|   Microchip Technology Inc.
|   PolarFire IBIS Model
[IBIS ver]   5.0
[File name]   polarfire_dio.ibs
[File Rev]   1.4
[Date]   Tue Jun 20 2023
[Source] Simulated Models ONLY.
   All data is based on Spice simulation. All performed at Microchip Technology Inc..
[Notes]  IBIS file for dedicated I/O Standards.
   The package parasitics of various package types are given.
   Uncomment the appropriate package before simulations.
   Revision History:
   Rev 1.4: 20-Jun-2023
   - Updated Vinl and Vinh values of LVPECL_33,MIPI_25,MIPI_33 receivers
   Rev 1.3: 23-May-2022
   - REFCLK buffers mapped to the VDD_XCVR_CLK supply in [Pin Mapping] section
   - Added MPF050 device with RLC package data in [Package] section
   - Added RLC package type of FCG784N for MPF300T device
   - Update RLC package data for 100T/200T/300T/500T devices
   Rev 1.2: 20-Sept-2021
   - Addition of LVDS ODT models
   Rev 1.1: 29-oct-2018
   - Fixed Power Clamp and Gnd Clamp data of standards
   LVTTL_33_ODT-OFF_HYST-OFF_refclk and LVCMOS25_25_ODT-75_HYST-ON_refclk
   - Added one supply pin in [pin] section
   - Added pin description in [Pin] section
   - Added [Pin Mapping] section
[Disclaimer] This information is for board design considerations.
   Simulation based V/I curves contained in this model file are
   considered preliminary until verified against bench
   measurements. Maximum currents may vary from part to part but
   should not exceed maximum I/V curves provided in this model file.
[Copyright]  (c) 2023, Microchip Technology Inc., All Rights Reserved.
| ADDITIONAL NOTES
| The naming conventions used in the signal_name/model_name are as follows:
| HYST-#  - Hysteresis setting,OFF or ON represented by #
| ODT-#   - Series on-die termination, impedance value represented by #
| #_I   - Refers to input models ,  model name represented by #
| #_O   - Refers to output models , model name represented by #
| #_IO   - Refers to Input/Output models,  model name represented by #
| IBIS MODEL CHECKLIST
| Microchip Technology Inc. is dedicated to releasing quality IBIS models to customers.
| The following items have been
| verified for this IBIS model before release:
| 1)  Checked IBIS model by the golden parser ibischk5 [Complete]
| 2)  Ensured no errors reported by golden parser
|   for the IBIS model [Complete]
| 3)  Defined Vinl and Vinh for receivers [Complete]
| 4)  Defined Standard Load and Vmeas values for drivers [Complete]
| 5)  Defined overshoots for drivers and receivers [NA]
| 6)  Validated Ramp Values[]
| 7)  Defined V-T Tables for all output drivers [Complete]
| 8)  Validated [Diff Pins] [NA]
| 9)  Verified Package Parasitics [Complete]
| 10) Defined Standard Load Parameters and Specifications
|   for waveforms [Complete]
| 11) Defined and Validate Pin mappings [Complete]
| 12) Verified Ccomp Value []
| 13) Visually Inspected I-V Curves and V-T Tables  [Complete]
| 14) Presented Typ/Min/Max Values in the correct order for
|   all tables and parameters [Complete]
| 15) Simulated all output models with standard load and
|   switching through Vmeas [Complete]
| 16) Simulated all receiver models  [Complete]
| 17) Validated Models selectors. [Complete]
| 18) Visually inspected Spice and IBIS correlation for
|   a) Typical VT Curves [Complete]
|   b) Minimum VT Curves [Complete]
|   c) Maximum VT Curves [Complete]
| 19) Visually inspected Silicon and IBIS correlation
|   a) Typical IV Pull UP/ Pull Down Curves []
|   b) Minimum IV Pull UP/ Pull Down Curves []
|   c) Maximum IV Pull UP/ Pull Down Curves []
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[Component]   PolarFire
[Manufacturer]   Microchip Technology Inc.
[Package]
|   typ   min   max
|MPF050T/TL/TLS/TS
|R_pkg   0.204   NA   NA   | MPF050T/TL/TLS/TS-FCSG325
|L_pkg   1.608nH   NA   NA   | MPF050T/TL/TLS/TS-FCSG325
|C_pkg   0.803pF   NA   NA   | MPF050T/TL/TLS/TS-FCSG325
|R_pkg   0.570   NA   NA   | MPF050T/TL/TLS/TS-FCVG484
|L_pkg   3.557nH   NA   NA   | MPF050T/TL/TLS/TS-FCVG484
|C_pkg   1.663pF   NA   NA   | MPF050T/TL/TLS/TS-FCVG484
|MPF100T/TL/TLS/TS
|R_pkg   0.253   NA   NA   | MPF100T/TL/TLS/TS-FCSG325
|L_pkg   1.920nH   NA   NA   | MPF100T/TL/TLS/TS-FCSG325
|C_pkg   0.703pF   NA   NA   | MPF100T/TL/TLS/TS-FCSG325
|R_pkg   0.628   NA   NA   | MPF100T/TL/TLS/TS-FCG484
|L_pkg   4.759nH   NA   NA   | MPF100T/TL/TLS/TS-FCG484
|C_pkg   2.176pF   NA   NA   | MPF100T/TL/TLS/TS-FCG484
|R_pkg   0.355   NA   NA   | MPF100T/TL/TLS/TS-FCVG484
|L_pkg   2.999nH   NA   NA   | MPF100T/TL/TLS/TS-FCVG484
|C_pkg   1.416pF   NA   NA   | MPF100T/TL/TLS/TS-FCVG484
|MPF200T/TL/TLS/TS
|R_pkg   0.316   NA   NA   | MPF200T/TL/TLS/TS-FCSG325
|L_pkg   2.423nH   NA   NA   | MPF200T/TL/TLS/TS-FCSG325
|C_pkg   0.844pF   NA   NA   | MPF200T/TL/TLS/TS-FCSG325
|R_pkg   0.518   NA   NA   | MPF200T/TL/TLS/TS-FCG484
|L_pkg   4.022nH   NA   NA   | MPF200T/TL/TLS/TS-FCG484
|C_pkg   1.858pF   NA   NA   | MPF200T/TL/TLS/TS-FCG484
|R_pkg   0.603   NA   NA   | MPF200T/TL/TLS/TS-FCVG484
|L_pkg   3.944nH   NA   NA   | MPF200T/TL/TLS/TS-FCVG484
|C_pkg   1.558pF   NA   NA   | MPF200T/TL/TLS/TS-FCVG484
|R_pkg   0.374   NA   NA   | MPF200T/TL/TLS/TS-FCSG536
|L_pkg   3.833nH   NA   NA   | MPF200T/TL/TLS/TS-FCSG536
|C_pkg   0.996pF   NA   NA   | MPF200T/TL/TLS/TS-FCSG536
|R_pkg   0.444   NA   NA   | MPF200T/TL/TLS/TS-FCG784
|L_pkg   3.672nH   NA   NA   | MPF200T/TL/TLS/TS-FCG784
|C_pkg   1.699pF   NA   NA   | MPF200T/TL/TLS/TS-FCG784
|MPF300T/TL/TLS/TS
|R_pkg   0.228   NA   NA   | MPF300T/TL/TLS/TS-FCG484
|L_pkg   2.178nH   NA   NA   | MPF300T/TL/TLS/TS-FCG484
|C_pkg   1.408pF   NA   NA   | MPF300T/TL/TLS/TS-FCG484
|R_pkg   0.661   NA   NA   | MPF300T/TL/TLS/TS-FCVG484
|L_pkg   4.585nH   NA   NA   | MPF300T/TL/TLS/TS-FCVG484
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R_pkg   0.735   NA   NA   | MPF300T/TL/TLS/TS-FCG1152
L_pkg   5.088nH   NA   NA   | MPF300T/TL/TLS/TS-FCG1152
C_pkg   2.163pF   NA   NA   | MPF300T/TL/TLS/TS-FCG1152
|MPF500T/TL/TLS/TS
|R_pkg   0.522   NA   NA   | MPF500T/TL/TLS/TS-FCG784
|L_pkg   3.540nH   NA   NA   | MPF500T/TL/TLS/TS-FCG784
|C_pkg   1.604pF   NA   NA   | MPF500T/TL/TLS/TS-FCG784
|R_pkg   0.594   NA   NA   | MPF500T/TL/TLS/TS-FCG1152
|L_pkg   3.914nH   NA   NA   | MPF500T/TL/TLS/TS-FCG1152
|C_pkg   1.587pF   NA   NA   | MPF500T/TL/TLS/TS-FCG1152
| End Header
| The PIN numbers given below are examples. They do not correspond to
| device pin numbers.
[Pin]   signal_name   model_name   R_pin   L_pin   C_pin
| SPI signals
1   sc_spi_sck   LVCMOS_iobuf_dio
2   sc_spi_ss   LVCMOS_iobuf_dio
3   sc_spi_sdo   LVCMOS_obuf_dio
| JTAG signals
4   jtag_tdo   LVCMOS_obuf_dio
5   jtag_tms   LVCMOS_ibuf_pullup_dio
6   jtag_tdi   LVCMOS_ibuf_pullup_dio
7   jtag_tck   LVCMOS_ibuf_dio
8   jtag_trstb   LVCMOS_ibuf_pullup_dio
| Device Reset (DEVRST_N)
9   devrst_b   LVCMOS_ibuf_pullup_dio
| UNUSED
10   sc_exit_flash_freeze   LVCMOS_ibuf_pullup_dio
| SPI signals
11   sc_spi_sdi   LVCMOS_ibuf_dio
12   sc_io_cfg_interface   LVCMOS_ibuf_dio
13   sc_io_cfg_flash   LVCMOS_ibuf_dio
| SERDES REFCLK
14   ref_clk   ref_clk_inputs
| Power Supplies
15   VDDI   POWER
16   VDD_XCVR_CLK   POWER
17   VSS   GND
| SERDES REFCLK_DIFF
18P   ref_clk_diff_ODT_OFF_P   ref_clk_inputs_DIFF_ODT_OFF
18N   ref_clk_diff_ODT_OFF_N   ref_clk_inputs_DIFF_ODT_OFF
19P   ref_clk_diff_ODT_ON_33_P   ref_clk_inputs_diff_ODT_ON_33
19N   ref_clk_diff_ODT_ON_33_N   ref_clk_inputs_diff_ODT_ON_33
20P   ref_clk_diff_ODT_ON_25_P   ref_clk_inputs_diff_ODT_ON_25
20N   ref_clk_diff_ODT_ON_25_N   ref_clk_inputs_diff_ODT_ON_25
[Pin Mapping]   pulldown_ref   pullup_ref   gnd_clamp_ref   power_clamp_ref ext_ref
1   VSS   VDDI   VSS   VDDI
2   VSS   VDDI   VSS   VDDI
3   VSS   VDDI   VSS   VDDI
4   VSS   VDDI   VSS   VDDI
5   VSS   VDDI   VSS   VDDI
6   VSS   VDDI   VSS   VDDI
7   VSS   VDDI   VSS   VDDI
8   VSS   VDDI   VSS   VDDI
9   VSS   VDDI   VSS   VDDI
10   VSS   VDDI   VSS   VDDI
11   VSS   VDDI   VSS   VDDI
12   VSS   VDDI   VSS   VDDI
13   VSS   VDDI   VSS   VDDI
14   VSS   VDD_XCVR_CLK   VSS   VDD_XCVR_CLK
15   NC   VDDI
16   NC   VDD_XCVR_CLK
17   VSS   NC
18P   VSS   VDD_XCVR_CLK   VSS   VDD_XCVR_CLK
18N   VSS   VDD_XCVR_CLK   VSS   VDD_XCVR_CLK
19P   VSS   VDD_XCVR_CLK   VSS   VDD_XCVR_CLK
19N   VSS   VDD_XCVR_CLK   VSS   VDD_XCVR_CLK
20P   VSS   VDD_XCVR_CLK   VSS   VDD_XCVR_CLK
20N   VSS   VDD_XCVR_CLK   VSS   VDD_XCVR_CLK
[Diff Pin]   inv_pin   vdiff   tdelay_typ   tdelay_min   tdelay_max
18P   18N   100mV   0   0   0
19P   19N   100mV   0   0   0
20P   20N   100mV   0   0   0
[Series Pin Mapping]   pin_2   model_name   function_table_group
19P   19N   ODT_33_TERM_100
20P   20N   ODT_25_TERM_100
|   Model Selector
[Model Selector]   LVCMOS_iobuf_dio
LVCMOS_33_HYST-ON_DIO_IO   3.3V I/O hysteresis ON
LVCMOS_25_HYST-ON_DIO_IO   2.5V I/O hysteresis ON
LVCMOS_18_HYST-ON_DIO_IO   1.8V I/O hysteresis ON
[Model Selector]   LVCMOS_obuf_dio
LVCMOS_33_HYST-OFF_DIO_O   3.3V Output hysteresis OFF
LVCMOS_25_HYST-OFF_DIO_O   2.5V Output hysteresis OFF
LVCMOS_18_HYST-OFF_DIO_O   1.8V Output hysteresis OFF
[Model Selector]   LVCMOS_ibuf_pullup_dio
LVCMOS_33_PM_HYST-ON_DIO_I   3.3V Input weak pullup hysteresis ON
LVCMOS_25_PM_HYST-ON_DIO_I   2.5V Input weak pullup hysteresis ON
LVCMOS_18_PM_DIO_I   1.8V Input weak pullup
[Model Selector]   LVCMOS_ibuf_dio
LVCMOS_33_HYST-ON_DIO_I   3.3V Input hysteresis ON
LVCMOS_25_HYST-ON_DIO_I   2.5V Input hysteresis ON
LVCMOS_18_DIO_I   1.8V Input
[Model Selector]   ref_clk_inputs
LVTTL_33_ODT-OFF_HYST-ON_refclk   3.3V LVTTL Standard
LVTTL_25_ODT-OFF_HYST-ON_refclk   2.5V LVTTL Standard
LVTTL_33_ODT-75_HYST-ON_refclk   3.3V LVTTL Standard
LVTTL_25_ODT-75_HYST-ON_refclk   2.5V LVTTL Standard
LVTTL_33_ODT-150_HYST-ON_refclk   3.3V LVTTL Standard
LVTTL_25_ODT-150_HYST-ON_refclk   2.5V LVTTL Standard
LVTTL_33_ODT-OFF_HYST-OFF_refclk   3.3V LVTTL Standard
LVTTL_25_ODT-OFF_HYST-OFF_refclk   2.5V LVTTL Standard
LVTTL_33_ODT-75_HYST-OFF_refclk   3.3V LVTTL Standard
LVTTL_25_ODT-75_HYST-OFF_refclk   2.5V LVTTL Standard
LVTTL_33_ODT-150_HYST-OFF_refclk   3.3V LVTTL Standard
LVTTL_25_ODT-150_HYST-OFF_refclk   2.5V LVTTL Standard
LVCMOS33_33_ODT-OFF_HYST-ON_refclk   3.3V LVCMOS33 Standard
LVCMOS33_25_ODT-OFF_HYST-ON_refclk   2.5V LVCMOS33 Standard
LVCMOS33_33_ODT-75_HYST-ON_refclk   3.3V LVCMOS33 Standard
LVCMOS33_25_ODT-75_HYST-ON_refclk   2.5V LVCMOS33 Standard
LVCMOS33_33_ODT-150_HYST-ON_refclk   3.3V LVCMOS33 Standard
LVCMOS33_25_ODT-150_HYST-ON_refclk   2.5V LVCMOS33 Standard
LVCMOS33_33_ODT-OFF_HYST-OFF_refclk   3.3V LVCMOS33 Standard
LVCMOS33_25_ODT-OFF_HYST-OFF_refclk   2.5V LVCMOS33 Standard
LVCMOS33_33_ODT-75_HYST-OFF_refclk   3.3V LVCMOS33 Standard
LVCMOS33_25_ODT-75_HYST-OFF_refclk   2.5V LVCMOS33 Standard
LVCMOS33_33_ODT-150_HYST-OFF_refclk   3.3V LVCMOS33 Standard
LVCMOS33_25_ODT-150_HYST-OFF_refclk   2.5V LVCMOS33 Standard
LVCMOS25_33_ODT-OFF_HYST-ON_refclk   3.3V LVCMOS25 Standard
LVCMOS25_25_ODT-OFF_HYST-ON_refclk   2.5V LVCMOS25 Standard
LVCMOS25_33_ODT-75_HYST-ON_refclk   3.3V LVCMOS25 Standard
LVCMOS25_25_ODT-75_HYST-ON_refclk   2.5V LVCMOS25 Standard
LVCMOS25_33_ODT-150_HYST-ON_refclk   3.3V LVCMOS25 Standard
LVCMOS25_25_ODT-150_HYST-ON_refclk   2.5V LVCMOS25 Standard
LVCMOS25_33_ODT-OFF_HYST-OFF_refclk   3.3V LVCMOS25 Standard
LVCMOS25_25_ODT-OFF_HYST-OFF_refclk   2.5V LVCMOS25 Standard
LVCMOS25_33_ODT-75_HYST-OFF_refclk   3.3V LVCMOS25 Standard
LVCMOS25_25_ODT-75_HYST-OFF_refclk   2.5V LVCMOS25 Standard
LVCMOS25_33_ODT-150_HYST-OFF_refclk   3.3V LVCMOS25 Standard
LVCMOS25_25_ODT-150_HYST-OFF_refclk   2.5V LVCMOS25 Standard
LVCMOS18_18_ODT-OFF_HYST-ON_refclk   1.8V LVCMOS18 Standard
LVCMOS18_25_ODT-OFF_HYST-ON_refclk   2.5V LVCMOS18 Standard
LVCMOS18_18_ODT-75_HYST-ON_refclk   1.8V LVCMOS18 Standard
LVCMOS18_25_ODT-75_HYST-ON_refclk   2.5V LVCMOS18 Standard
LVCMOS18_18_ODT-150_HYST-ON_refclk   1.8V LVCMOS18 Standard
LVCMOS18_25_ODT-150_HYST-ON_refclk   2.5V LVCMOS18 Standard
LVCMOS18_18_ODT-OFF_HYST-OFF_refclk   1.8V LVCMOS18 Standard
LVCMOS18_25_ODT-OFF_HYST-OFF_refclk   2.5V LVCMOS18 Standard
LVCMOS18_18_ODT-75_HYST-OFF_refclk   1.8V LVCMOS18 Standard
LVCMOS18_25_ODT-75_HYST-OFF_refclk   2.5V LVCMOS18 Standard
LVCMOS18_18_ODT-150_HYST-OFF_refclk   1.8V LVCMOS18 Standard
LVCMOS18_25_ODT-150_HYST-OFF_refclk   2.5V LVCMOS18 Standard
SSTL25I_25_ODT-OFF_HYST-ON_refclk   2.5V SSTL25I Standard
SSTL25I_25_ODT-OFF_HYST-OFF_refclk   2.5V SSTL25I Standard
SSTL25II_25_ODT-OFF_HYST-ON_refclk   2.5V SSTL25II Standard
SSTL25II_25_ODT-OFF_HYST-OFF_refclk   2.5V SSTL25II Standard
SSTL18I_25_ODT-OFF_HYST-ON_refclk   2.5V SSTL18I Standard
SSTL18I_25_ODT-OFF_HYST-OFF_refclk   2.5V SSTL18I Standard
SSTL18II_25_ODT-OFF_HYST-ON_refclk   2.5V SSTL18II Standard
SSTL18II_25_ODT-OFF_HYST-OFF_refclk   2.5V SSTL18II Standard
SSTL25DI_25_ODT-OFF_HYST-ON_N_refclk   2.5V SSTL25DI Standard
SSTL25DI_25_ODT-OFF_HYST-ON_P_refclk   2.5V SSTL25DI Standard
SSTL25DI_25_ODT-OFF_HYST-OFF_N_refclk   2.5V SSTL25DI Standard
SSTL25DI_25_ODT-OFF_HYST-OFF_P_refclk   2.5V SSTL25DI Standard
SSTL25DII_25_ODT-OFF_HYST-ON_N_refclk   2.5V SSTL25DII Standard
SSTL25DII_25_ODT-OFF_HYST-ON_P_refclk   2.5V SSTL25DII Standard
SSTL25DII_25_ODT-OFF_HYST-OFF_N_refclk   2.5V SSTL25DII Standard
SSTL25DII_25_ODT-OFF_HYST-OFF_P_refclk   2.5V SSTL25DII Standard
SSTL18DI_25_ODT-OFF_HYST-ON_N_refclk   2.5V SSTL18DI Standard
SSTL18DI_25_ODT-OFF_HYST-ON_P_refclk   2.5V SSTL18DI Standard
SSTL18DI_25_ODT-OFF_HYST-OFF_N_refclk   2.5V SSTL18DI Standard
SSTL18DI_25_ODT-OFF_HYST-OFF_P_refclk   2.5V SSTL18DI Standard
SSTL18DII_25_ODT-OFF_HYST-ON_N_refclk   2.5V SSTL18DII Standard
SSTL18DII_25_ODT-OFF_HYST-ON_P_refclk   2.5V SSTL18DII Standard
SSTL18DII_25_ODT-OFF_HYST-OFF_N_refclk   2.5V SSTL18DII Standard
SSTL18DII_25_ODT-OFF_HYST-OFF_P_refclk   2.5V SSTL18DII Standard
HSUL18I_25_ODT-OFF_HYST-ON_refclk   2.5V HSUL18I Standard
HSUL18I_25_ODT-OFF_HYST-OFF_refclk   2.5V HSUL18I Standard
HSUL18II_25_ODT-OFF_HYST-ON_refclk   2.5V HSUL18II Standard
HSUL18II_25_ODT-OFF_HYST-OFF_refclk   2.5V HSUL18II Standard
HSUL18DI_25_ODT-OFF_HYST-ON_N_refclk   2.5V HSUL18DI Standard
HSUL18DI_25_ODT-OFF_HYST-ON_P_refclk   2.5V HSUL18DI Standard
HSUL18DI_25_ODT-OFF_HYST-OFF_N_refclk   2.5V HSUL18DI Standard
HSUL18DI_25_ODT-OFF_HYST-OFF_P_refclk   2.5V HSUL18DI Standard
HSUL18DII_25_ODT-OFF_HYST-ON_N_refclk   2.5V HSUL18DII Standard
HSUL18DII_25_ODT-OFF_HYST-ON_P_refclk   2.5V HSUL18DII Standard
HSUL18DII_25_ODT-OFF_HYST-OFF_N_refclk   2.5V HSUL18DII Standard
HSUL18DII_25_ODT-OFF_HYST-OFF_P_refclk   2.5V HSUL18DII Standard
[Model Selector]   ref_clk_inputs_DIFF_ODT_OFF
LVDS_33_ODT-OFF_HYST-ON_N_refclk   3.3V LVDS Standard
LVDS_33_ODT-OFF_HYST-ON_P_refclk   3.3V LVDS Standard
LVDS_25_ODT-OFF_HYST-ON_N_refclk   2.5V LVDS Standard
LVDS_25_ODT-OFF_HYST-ON_P_refclk   2.5V LVDS Standard
LVDS_33_ODT-OFF_HYST-OFF_N_refclk   3.3V LVDS Standard
LVDS_33_ODT-OFF_HYST-OFF_P_refclk   3.3V LVDS Standard
LVDS_25_ODT-OFF_HYST-OFF_N_refclk   2.5V LVDS Standard
LVDS_25_ODT-OFF_HYST-OFF_P_refclk   2.5V LVDS Standard
RSDS_33_ODT-OFF_HYST-ON_N_refclk   3.3V RSDS Standard
RSDS_33_ODT-OFF_HYST-ON_P_refclk   3.3V RSDS Standard
RSDS_25_ODT-OFF_HYST-ON_N_refclk   2.5V RSDS Standard
RSDS_25_ODT-OFF_HYST-ON_P_refclk   2.5V RSDS Standard
RSDS_33_ODT-OFF_HYST-OFF_N_refclk   3.3V RSDS Standard
RSDS_33_ODT-OFF_HYST-OFF_P_refclk   3.3V RSDS Standard
RSDS_25_ODT-OFF_HYST-OFF_N_refclk   2.5V RSDS Standard
RSDS_25_ODT-OFF_HYST-OFF_P_refclk   2.5V RSDS Standard
MINILVDS_33_ODT-OFF_HYST-ON_N_refclk   3.3V MINILVDS Standard
MINILVDS_33_ODT-OFF_HYST-ON_P_refclk   3.3V MINILVDS Standard
MINILVDS_25_ODT-OFF_HYST-ON_N_refclk   2.5V MINILVDS Standard
MINILVDS_25_ODT-OFF_HYST-ON_P_refclk   2.5V MINILVDS Standard
MINILVDS_33_ODT-OFF_HYST-OFF_N_refclk   3.3V MINILVDS Standard
MINILVDS_33_ODT-OFF_HYST-OFF_P_refclk   3.3V MINILVDS Standard
MINILVDS_25_ODT-OFF_HYST-OFF_N_refclk   2.5V MINILVDS Standard
MINILVDS_25_ODT-OFF_HYST-OFF_P_refclk   2.5V MINILVDS Standard
SUBLVDS_33_ODT-OFF_HYST-ON_N_refclk   3.3V SUBLVDS Standard
SUBLVDS_33_ODT-OFF_HYST-ON_P_refclk   3.3V SUBLVDS Standard
SUBLVDS_25_ODT-OFF_HYST-ON_N_refclk   2.5V SUBLVDS Standard
SUBLVDS_25_ODT-OFF_HYST-ON_P_refclk   2.5V SUBLVDS Standard
SUBLVDS_33_ODT-OFF_HYST-OFF_N_refclk   3.3V SUBLVDS Standard
SUBLVDS_33_ODT-OFF_HYST-OFF_P_refclk   3.3V SUBLVDS Standard
SUBLVDS_25_ODT-OFF_HYST-OFF_N_refclk   2.5V SUBLVDS Standard
SUBLVDS_25_ODT-OFF_HYST-OFF_P_refclk   2.5V SUBLVDS Standard
PPDS_33_ODT-OFF_HYST-ON_N_refclk   3.3V PPDS Standard
PPDS_33_ODT-OFF_HYST-ON_P_refclk   3.3V PPDS Standard
PPDS_25_ODT-OFF_HYST-ON_N_refclk   2.5V PPDS Standard
PPDS_25_ODT-OFF_HYST-ON_P_refclk   2.5V PPDS Standard
PPDS_33_ODT-OFF_HYST-OFF_N_refclk   3.3V PPDS Standard
PPDS_33_ODT-OFF_HYST-OFF_P_refclk   3.3V PPDS Standard
PPDS_25_ODT-OFF_HYST-OFF_N_refclk   2.5V PPDS Standard
PPDS_25_ODT-OFF_HYST-OFF_P_refclk   2.5V PPDS Standard
SLVS_33_ODT-OFF_HYST-ON_N_refclk   3.3V SLVS Standard
SLVS_33_ODT-OFF_HYST-ON_P_refclk   3.3V SLVS Standard
SLVS_25_ODT-OFF_HYST-ON_N_refclk   2.5V SLVS Standard
SLVS_25_ODT-OFF_HYST-ON_P_refclk   2.5V SLVS Standard
SLVS_33_ODT-OFF_HYST-OFF_N_refclk   3.3V SLVS Standard
SLVS_33_ODT-OFF_HYST-OFF_P_refclk   3.3V SLVS Standard
SLVS_25_ODT-OFF_HYST-OFF_N_refclk   2.5V SLVS Standard
SLVS_25_ODT-OFF_HYST-OFF_P_refclk   2.5V SLVS Standard
HCSL_33_ODT-OFF_HYST-ON_N_refclk   3.3V HCSL Standard
HCSL_33_ODT-OFF_HYST-ON_P_refclk   3.3V HCSL Standard
HCSL_25_ODT-OFF_HYST-ON_N_refclk   2.5V HCSL Standard
HCSL_25_ODT-OFF_HYST-ON_P_refclk   2.5V HCSL Standard
HCSL_33_ODT-OFF_HYST-OFF_N_refclk   3.3V HCSL Standard
HCSL_33_ODT-OFF_HYST-OFF_P_refclk   3.3V HCSL Standard
HCSL_25_ODT-OFF_HYST-OFF_N_refclk   2.5V HCSL Standard
HCSL_25_ODT-OFF_HYST-OFF_P_refclk   2.5V HCSL Standard
MLVDS_33_ODT-OFF_HYST-ON_N_refclk   3.3V MLVDS Standard
MLVDS_33_ODT-OFF_HYST-ON_P_refclk   3.3V MLVDS Standard
MLVDS_25_ODT-OFF_HYST-ON_N_refclk   2.5V MLVDS Standard
MLVDS_25_ODT-OFF_HYST-ON_P_refclk   2.5V MLVDS Standard
MLVDS_33_ODT-OFF_HYST-OFF_N_refclk   3.3V MLVDS Standard
MLVDS_33_ODT-OFF_HYST-OFF_P_refclk   3.3V MLVDS Standard
MLVDS_25_ODT-OFF_HYST-OFF_N_refclk   2.5V MLVDS Standard
MLVDS_25_ODT-OFF_HYST-OFF_P_refclk   2.5V MLVDS Standard
LVPECL_33_ODT-OFF_HYST-ON_N_refclk   3.3V LVPECL Standard
LVPECL_33_ODT-OFF_HYST-ON_P_refclk   3.3V LVPECL Standard
LVPECL_33_ODT-OFF_HYST-OFF_N_refclk   3.3V LVPECL Standard
LVPECL_33_ODT-OFF_HYST-OFF_P_refclk   3.3V LVPECL Standard
MIPI_25_ODT-OFF_HYST-ON_N_refclk   2.5V MIPI Standard
MIPI_25_ODT-OFF_HYST-ON_P_refclk   2.5V MIPI Standard
MIPI_33_ODT-OFF_HYST-ON_N_refclk   3.3V MIPI Standard
MIPI_33_ODT-OFF_HYST-ON_P_refclk   3.3V MIPI Standard
MIPI_25_ODT-OFF_HYST-OFF_N_refclk   2.5V MIPI Standard
MIPI_25_ODT-OFF_HYST-OFF_P_refclk   2.5V MIPI Standard
MIPI_33_ODT-OFF_HYST-OFF_N_refclk   3.3V MIPI Standard
MIPI_33_ODT-OFF_HYST-OFF_P_refclk   3.3V MIPI Standard
[Model Selector]   ref_clk_inputs_diff_ODT_ON_33
LVDS_33_ODT-OFF_HYST-ON_N_refclk   3.3V LVDS Standard
LVDS_33_ODT-OFF_HYST-ON_P_refclk   3.3V LVDS Standard
LVDS_33_ODT-OFF_HYST-OFF_N_refclk   3.3V LVDS Standard
LVDS_33_ODT-OFF_HYST-OFF_P_refclk   3.3V LVDS Standard
RSDS_33_ODT-OFF_HYST-ON_N_refclk   3.3V RSDS Standard
RSDS_33_ODT-OFF_HYST-ON_P_refclk   3.3V RSDS Standard
RSDS_33_ODT-OFF_HYST-OFF_N_refclk   3.3V RSDS Standard
RSDS_33_ODT-OFF_HYST-OFF_P_refclk   3.3V RSDS Standard
MINILVDS_33_ODT-OFF_HYST-ON_N_refclk   3.3V MINILVDS Standard
MINILVDS_33_ODT-OFF_HYST-ON_P_refclk   3.3V MINILVDS Standard
MINILVDS_33_ODT-OFF_HYST-OFF_N_refclk   3.3V MINILVDS Standard
MINILVDS_33_ODT-OFF_HYST-OFF_P_refclk   3.3V MINILVDS Standard
SUBLVDS_33_ODT-OFF_HYST-ON_N_refclk   3.3V SUBLVDS Standard
SUBLVDS_33_ODT-OFF_HYST-ON_P_refclk   3.3V SUBLVDS Standard
SUBLVDS_33_ODT-OFF_HYST-OFF_N_refclk   3.3V SUBLVDS Standard
SUBLVDS_33_ODT-OFF_HYST-OFF_P_refclk   3.3V SUBLVDS Standard
PPDS_33_ODT-OFF_HYST-ON_N_refclk   3.3V PPDS Standard
PPDS_33_ODT-OFF_HYST-ON_P_refclk   3.3V PPDS Standard
PPDS_33_ODT-OFF_HYST-OFF_N_refclk   3.3V PPDS Standard
PPDS_33_ODT-OFF_HYST-OFF_P_refclk   3.3V PPDS Standard
SLVS_33_ODT-OFF_HYST-ON_N_refclk   3.3V SLVS Standard
SLVS_33_ODT-OFF_HYST-ON_P_refclk   3.3V SLVS Standard
SLVS_33_ODT-OFF_HYST-OFF_N_refclk   3.3V SLVS Standard
SLVS_33_ODT-OFF_HYST-OFF_P_refclk   3.3V SLVS Standard
HCSL_33_ODT-OFF_HYST-ON_N_refclk   3.3V HCSL Standard
HCSL_33_ODT-OFF_HYST-ON_P_refclk   3.3V HCSL Standard
HCSL_33_ODT-OFF_HYST-OFF_N_refclk   3.3V HCSL Standard
HCSL_33_ODT-OFF_HYST-OFF_P_refclk   3.3V HCSL Standard
MLVDS_33_ODT-OFF_HYST-ON_N_refclk   3.3V MLVDS Standard
MLVDS_33_ODT-OFF_HYST-ON_P_refclk   3.3V MLVDS Standard
MLVDS_33_ODT-OFF_HYST-OFF_N_refclk   3.3V MLVDS Standard
MLVDS_33_ODT-OFF_HYST-OFF_P_refclk   3.3V MLVDS Standard
LVPECL_33_ODT-OFF_HYST-ON_N_refclk   3.3V LVPECL Standard
LVPECL_33_ODT-OFF_HYST-ON_P_refclk   3.3V LVPECL Standard
LVPECL_33_ODT-OFF_HYST-OFF_N_refclk   3.3V LVPECL Standard
LVPECL_33_ODT-OFF_HYST-OFF_P_refclk   3.3V LVPECL Standard
MIPI_33_ODT-OFF_HYST-ON_N_refclk   3.3V MIPI Standard
MIPI_33_ODT-OFF_HYST-ON_P_refclk   3.3V MIPI Standard
MIPI_33_ODT-OFF_HYST-OFF_N_refclk   3.3V MIPI Standard
MIPI_33_ODT-OFF_HYST-OFF_P_refclk   3.3V MIPI Standard
[Model Selector]   ref_clk_inputs_diff_ODT_ON_25
LVDS_25_ODT-OFF_HYST-ON_N_refclk   2.5V LVDS Standard
LVDS_25_ODT-OFF_HYST-ON_P_refclk   2.5V LVDS Standard
LVDS_25_ODT-OFF_HYST-OFF_N_refclk   2.5V LVDS Standard
LVDS_25_ODT-OFF_HYST-OFF_P_refclk   2.5V LVDS Standard
RSDS_25_ODT-OFF_HYST-ON_N_refclk   2.5V RSDS Standard
RSDS_25_ODT-OFF_HYST-ON_P_refclk   2.5V RSDS Standard
RSDS_25_ODT-OFF_HYST-OFF_N_refclk   2.5V RSDS Standard
RSDS_25_ODT-OFF_HYST-OFF_P_refclk   2.5V RSDS Standard
MINILVDS_25_ODT-OFF_HYST-ON_N_refclk   2.5V MINILVDS Standard
MINILVDS_25_ODT-OFF_HYST-ON_P_refclk   2.5V MINILVDS Standard
MINILVDS_25_ODT-OFF_HYST-OFF_N_refclk   2.5V MINILVDS Standard
MINILVDS_25_ODT-OFF_HYST-OFF_P_refclk   2.5V MINILVDS Standard
SUBLVDS_25_ODT-OFF_HYST-ON_N_refclk   2.5V SUBLVDS Standard
SUBLVDS_25_ODT-OFF_HYST-ON_P_refclk   2.5V SUBLVDS Standard
SUBLVDS_25_ODT-OFF_HYST-OFF_N_refclk   2.5V SUBLVDS Standard
SUBLVDS_25_ODT-OFF_HYST-OFF_P_refclk   2.5V SUBLVDS Standard
PPDS_25_ODT-OFF_HYST-ON_N_refclk   2.5V PPDS Standard
PPDS_25_ODT-OFF_HYST-ON_P_refclk   2.5V PPDS Standard
PPDS_25_ODT-OFF_HYST-OFF_N_refclk   2.5V PPDS Standard
PPDS_25_ODT-OFF_HYST-OFF_P_refclk   2.5V PPDS Standard
SLVS_25_ODT-OFF_HYST-ON_N_refclk   2.5V SLVS Standard
SLVS_25_ODT-OFF_HYST-ON_P_refclk   2.5V SLVS Standard
SLVS_25_ODT-OFF_HYST-OFF_N_refclk   2.5V SLVS Standard
SLVS_25_ODT-OFF_HYST-OFF_P_refclk   2.5V SLVS Standard
HCSL_25_ODT-OFF_HYST-ON_N_refclk   2.5V HCSL Standard
HCSL_25_ODT-OFF_HYST-ON_P_refclk   2.5V HCSL Standard
HCSL_25_ODT-OFF_HYST-OFF_N_refclk   2.5V HCSL Standard
HCSL_25_ODT-OFF_HYST-OFF_P_refclk   2.5V HCSL Standard
MLVDS_25_ODT-OFF_HYST-ON_N_refclk   2.5V MLVDS Standard
MLVDS_25_ODT-OFF_HYST-ON_P_refclk   2.5V MLVDS Standard
MLVDS_25_ODT-OFF_HYST-OFF_N_refclk   2.5V MLVDS Standard
MLVDS_25_ODT-OFF_HYST-OFF_P_refclk   2.5V MLVDS Standard
MIPI_25_ODT-OFF_HYST-ON_N_refclk   2.5V MIPI Standard
MIPI_25_ODT-OFF_HYST-ON_P_refclk   2.5V MIPI Standard
MIPI_25_ODT-OFF_HYST-OFF_N_refclk   2.5V MIPI Standard
MIPI_25_ODT-OFF_HYST-OFF_P_refclk   2.5V MIPI Standard
|   Model  ODT_25_TERM_100
[Model]   ODT_25_TERM_100
Model_type   Series
Polarity   Non-Inverting
C_comp   5.210e-12   5.210e-12   5.520e-12
[Temperature Range]   25C   100C   -40C
[Voltage Range]   2.5V   2.375V   2.625V
[R Series]   100   80   125
| End [Model] ODT_25_TERM_100
|   Model  ODT_33_TERM_100
[Model]   ODT_33_TERM_100
Model_type   Series
Polarity   Non-Inverting
C_comp   5.210e-12   5.210e-12   5.520e-12
[Temperature Range]   25C   100C   -40C
[Voltage Range]   3.3V   3.135V   3.465V
[R Series]   100   80   125
| End [Model] ODT_33_TERM_100
| End [Component]
| Models and submodels in the file (174): LVCMOS_33_HYST-ON_DIO_IO (I/O), LVCMOS_25_HYST-ON_DIO_IO (I/O), LVCMOS_18_HYST-ON_DIO_IO (I/O), LVCMOS_33_HYST-OFF_DIO_O (Output), LVCMOS_25_HYST-OFF_DIO_O (Output), LVCMOS_18_HYST-OFF_DIO_O (Output), LVCMOS_33_PM_HYST-ON_DIO_I (Input), LVCMOS_25_PM_HYST-ON_DIO_I (Input), LVCMOS_18_PM_DIO_I (Input), LVCMOS_33_HYST-ON_DIO_I (Input), LVCMOS_25_HYST-ON_DIO_I (Input), LVCMOS_18_DIO_I (Input), LVTTL_33_ODT-OFF_HYST-ON_refclk (Input), LVTTL_25_ODT-OFF_HYST-ON_refclk (Input), LVTTL_33_ODT-75_HYST-ON_refclk (Input), LVTTL_25_ODT-75_HYST-ON_refclk (Input), LVTTL_33_ODT-150_HYST-ON_refclk (Input), LVTTL_25_ODT-150_HYST-ON_refclk (Input), LVTTL_33_ODT-OFF_HYST-OFF_refclk (Input), LVTTL_25_ODT-OFF_HYST-OFF_refclk (Input), LVTTL_33_ODT-75_HYST-OFF_refclk (Input), LVTTL_25_ODT-75_HYST-OFF_refclk (Input), LVTTL_33_ODT-150_HYST-OFF_refclk (Input), LVTTL_25_ODT-150_HYST-OFF_refclk (Input), LVCMOS33_33_ODT-OFF_HYST-ON_refclk (Input), LVCMOS33_25_ODT-OFF_HYST-ON_refclk (Input), LVCMOS33_33_ODT-75_HYST-ON_refclk (Input), LVCMOS33_25_ODT-75_HYST-ON_refclk (Input), LVCMOS33_33_ODT-150_HYST-ON_refclk (Input), LVCMOS33_25_ODT-150_HYST-ON_refclk (Input), LVCMOS33_33_ODT-OFF_HYST-OFF_refclk (Input), LVCMOS33_25_ODT-OFF_HYST-OFF_refclk (Input), LVCMOS33_33_ODT-75_HYST-OFF_refclk (Input), LVCMOS33_25_ODT-75_HYST-OFF_refclk (Input), LVCMOS33_33_ODT-150_HYST-OFF_refclk (Input), LVCMOS33_25_ODT-150_HYST-OFF_refclk (Input), LVCMOS25_33_ODT-OFF_HYST-ON_refclk (Input), LVCMOS25_25_ODT-OFF_HYST-ON_refclk (Input), LVCMOS25_33_ODT-75_HYST-ON_refclk (Input), LVCMOS25_25_ODT-75_HYST-ON_refclk (Input), LVCMOS25_33_ODT-150_HYST-ON_refclk (Input), LVCMOS25_25_ODT-150_HYST-ON_refclk (Input), LVCMOS25_33_ODT-OFF_HYST-OFF_refclk (Input), LVCMOS25_25_ODT-OFF_HYST-OFF_refclk (Input), LVCMOS25_33_ODT-75_HYST-OFF_refclk (Input), LVCMOS25_25_ODT-75_HYST-OFF_refclk (Input), LVCMOS25_33_ODT-150_HYST-OFF_refclk (Input), LVCMOS25_25_ODT-150_HYST-OFF_refclk (Input), LVCMOS18_18_ODT-OFF_HYST-ON_refclk (Input), LVCMOS18_25_ODT-OFF_HYST-ON_refclk (Input), LVCMOS18_18_ODT-75_HYST-ON_refclk (Input), LVCMOS18_25_ODT-75_HYST-ON_refclk (Input), LVCMOS18_18_ODT-150_HYST-ON_refclk (Input), LVCMOS18_25_ODT-150_HYST-ON_refclk (Input), LVCMOS18_18_ODT-OFF_HYST-OFF_refclk (Input), LVCMOS18_25_ODT-OFF_HYST-OFF_refclk (Input), LVCMOS18_18_ODT-75_HYST-OFF_refclk (Input), LVCMOS18_25_ODT-75_HYST-OFF_refclk (Input), LVCMOS18_18_ODT-150_HYST-OFF_refclk (Input), LVCMOS18_25_ODT-150_HYST-OFF_refclk (Input), SSTL25I_25_ODT-OFF_HYST-ON_refclk (Input), SSTL25I_25_ODT-OFF_HYST-OFF_refclk (Input), SSTL25II_25_ODT-OFF_HYST-ON_refclk (Input), SSTL25II_25_ODT-OFF_HYST-OFF_refclk (Input), SSTL18I_25_ODT-OFF_HYST-ON_refclk (Input), SSTL18I_25_ODT-OFF_HYST-OFF_refclk (Input), SSTL18II_25_ODT-OFF_HYST-ON_refclk (Input), SSTL18II_25_ODT-OFF_HYST-OFF_refclk (Input), HSUL18I_25_ODT-OFF_HYST-ON_refclk (Input), HSUL18I_25_ODT-OFF_HYST-OFF_refclk (Input), HSUL18II_25_ODT-OFF_HYST-ON_refclk (Input), HSUL18II_25_ODT-OFF_HYST-OFF_refclk (Input), LVDS_33_ODT-OFF_HYST-ON_N_refclk (Input), LVDS_33_ODT-OFF_HYST-ON_P_refclk (Input), LVDS_25_ODT-OFF_HYST-ON_N_refclk (Input), LVDS_25_ODT-OFF_HYST-ON_P_refclk (Input), LVDS_33_ODT-OFF_HYST-OFF_N_refclk (Input), LVDS_33_ODT-OFF_HYST-OFF_P_refclk (Input), LVDS_25_ODT-OFF_HYST-OFF_N_refclk (Input), LVDS_25_ODT-OFF_HYST-OFF_P_refclk (Input)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
